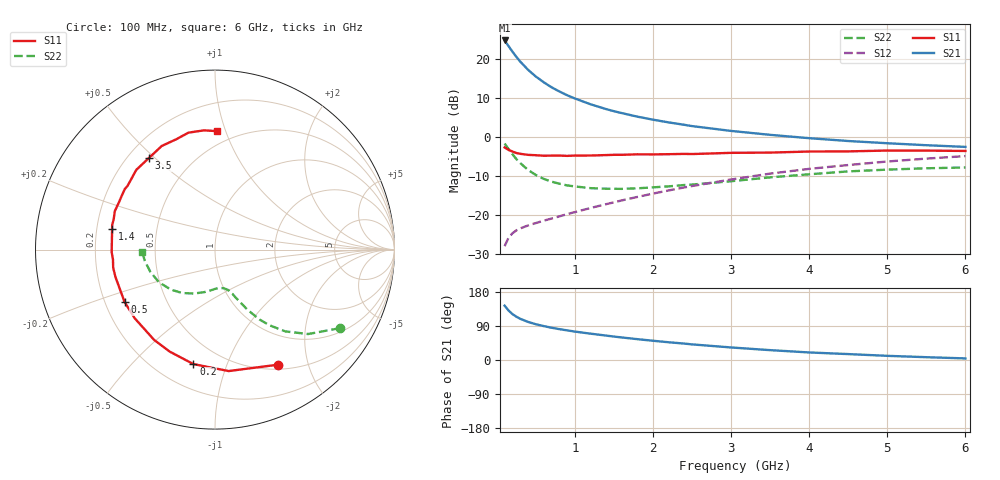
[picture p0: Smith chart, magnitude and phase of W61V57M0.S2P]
! SIEMENS Small Signal Semiconductors
! BFR193W
! Si NPN RF Bipolar Junction Transistor in SOT323
! VCE = 1.5 V  IC = 7 mA
! Common Emitter S-Parameters:  September  1992
# GHz  S  MA  R  50
!  f  S11  S21  S12  S22
! GHz  MAG  ANG  MAG  ANG  MAG  ANG  MAG  ANG
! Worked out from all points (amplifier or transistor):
!   28 points, 100 MHz to 6 GHz, reference 50 ohm
!   highest |S21| = 24.7 dB at 100 MHz (marker M1)
!   |S21| within 3 dB of that: start of sweep to 205.4 MHz
!   unconditionally stable (mu >= 1): 1.071 GHz to 2.641 GHz
!   at 300 MHz: K = 0.46, MSG = 21.4 dB, |S12| = -23.5 dB
!   at 1.5 GHz: K = 1.06, MAG = 10.2 dB, |S12| = -16.8 dB
!   at 6 GHz: K = 0.92, MSG = 1.2 dB, |S12| = -4.9 dB
!   S11 on the Smith chart (normalised r, x): 100 MHz: 0.56, -1.55; 200 MHz: 0.35, -0.77; 500 MHz: 0.28, -0.25; 1.4 GHz: 0.26, +0.09; 3.5 GHz: 0.28, +0.48; 6 GHz: 0.40, +0.94
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0.1  0.732 -61.1  17.19 143.4  0.0398 61.8  0.8217 -32.2
0.15  0.681 -83.6  14.55 130.7  0.051 53.6  0.7003 -42.2
0.2  0.6491 -100.7  12.37 121.2  0.0582 48.4  0.6013 -49.3
0.25  0.6217 -114.0  10.6 114.3  0.0634 45.6  0.52 -54.2
0.3  0.6068 -124.0  9.221 108.8  0.0672 44.0  0.4622 -57.5
0.4  0.5886 -139.5  7.231 100.5  0.0733 43.4  0.3773 -61.8
0.5  0.5821 -150.0  5.927 94.4  0.0787 44.3  0.3248 -64.4
0.6  0.5736 -158.2  5.015 89.5  0.0844 45.9  0.29 -66.8
0.7  0.5752 -164.5  4.322 85.2  0.0898 47.5  0.2672 -68.3
0.8  0.5762 -169.9  3.823 81.5  0.0958 49.3  0.2514 -70.2
0.9  0.5711 -174.5  3.417 78.2  0.1024 51.0  0.2391 -71.5
1  0.5758 -178.5  3.104 75.0  0.1087 52.6  0.2319 -73.3
1.2  0.577 174.6  2.617 69.5  0.1227 55.1  0.2203 -77.4
1.4  0.5846 168.7  2.268 64.4  0.1374 57.1  0.2167 -81.4
1.8  0.5979 159.0  1.816 55.0  0.17 59.7  0.2193 -90.1
2.2  0.6001 149.9  1.533 46.8  0.2059 60.4  0.2322 -98.3
2.5  0.6028 144.0  1.374 41.2  0.2346 60.2  0.2449 -104.5
3  0.6243 134.6  1.192 33.1  0.2846 58.3  0.2704 -115.2
3.5  0.6291 126.0  1.062 26.0  0.3383 55.2  0.3029 -126.9
4.5  0.6518 109.1  0.885 15.6  0.4359 46.7  0.3612 -149.7
5.5  0.6672 95.3  0.782 7.4  0.5267 37.2  0.396 -170.7
6  0.6601 88.9  0.744 4.2  0.5674 32.0  0.4055 -178.2
